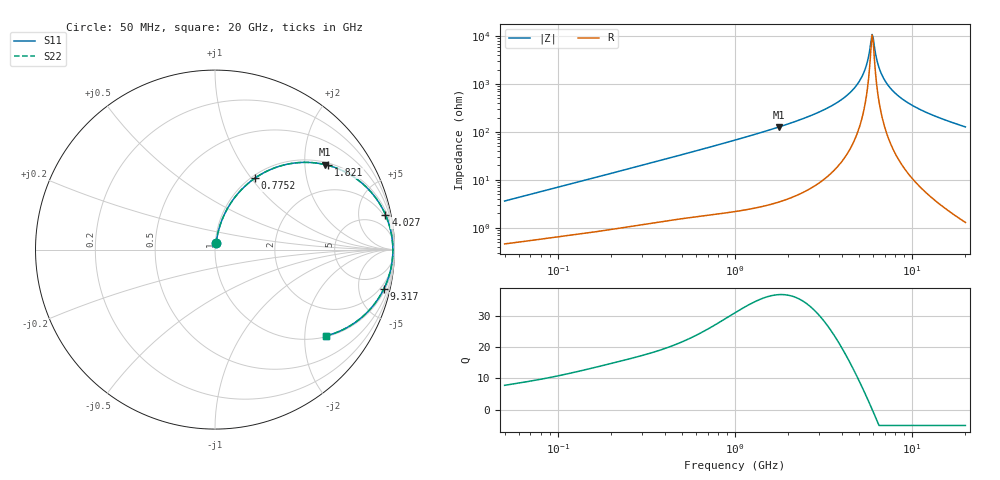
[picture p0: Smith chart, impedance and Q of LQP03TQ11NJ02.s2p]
!Murata Part Number: LQP03TQ11NJ02
!These Parameters are Measured in Series Mode Connection
!  o--[Z]--o
!Port1  Port2
!  o-------o
!Freq. Start=50[MHz] Stop=20[GHz], 401[Steps]
# Hz S RI R 50
!Freq.(Hz) S11(Real) S11(Imag) S21(Real) S21(Imag) S12(Real) S12(Imag) S22(Real) S22(Imag)
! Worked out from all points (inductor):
!   401 points, 50 MHz to 20 GHz, reference 50 ohm
!   read as one part in series: L = 11.4 nH near 51.52 MHz
!   highest Q = 36.7 at 1.767 GHz (marker M1), where L = 11.4 nH
!   self-resonance near 5.944 GHz
!   S11 on the Smith chart (normalised r, x): 50 MHz: 1.01, +0.07; 775.2 MHz: 1.04, +1.04; 1.821 GHz: 1.07, +2.63; 4.027 GHz: 1.49, +9.65; 9.317 GHz: 1.30, -8.44; 20 GHz: 1.03, -2.55
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5e7  0.00588 0.0356  0.9941 -0.0356  0.9941 -0.0356  0.00588 0.0356
1.364002e8  0.0162 0.0923  0.9838 -0.0923  0.9838 -0.0923  0.0162 0.0923
3.721004e8  0.07 0.23  0.93 -0.23  0.93 -0.23  0.07 0.23
7.751977e8  0.2215 0.3972  0.7785 -0.3972  0.7785 -0.3972  0.2215 0.3972
1e9  0.3194 0.4504  0.6806 -0.4504  0.6806 -0.4504  0.3194 0.4504
1.766834e9  0.6135 0.4735  0.3865 -0.4735  0.3865 -0.4735  0.6135 0.4735
1.820564e9  0.6299 0.4694  0.3701 -0.4694  0.3701 -0.4694  0.6299 0.4694
2.728004e9  0.8282 0.3621  0.1718 -0.3621  0.1718 -0.3621  0.8282 0.3621
4.026975e9  0.9498 0.1942  0.0502 -0.1942  0.0502 -0.1942  0.9498 0.1942
4.677679e9  0.9751 0.1215  0.0249 -0.1215  0.0249 -0.1215  0.9751 0.1215
5.194772e9  0.9857 0.0694  0.0143 -0.0694  0.0143 -0.0694  0.9857 0.0694
5.515528e9  0.9892 0.0393  0.0108 -0.0393  0.0108 -0.0393  0.9892 0.0393
5.856089e9  0.9909 0.00915  0.00915 -0.00915  0.00915 -0.00915  0.9909 0.00915
5.944466e9  0.991 0.0016  0.00903 -0.0016  0.00903 -0.0016  0.991 0.0016
6.125241e9  0.9909 -0.0135  0.00914 0.0135  0.00914 0.0135  0.9909 -0.0135
6.406762e9  0.9898 -0.0361  0.0102 0.0361  0.0102 0.0361  0.9898 -0.0361
6.601595e9  0.9885 -0.0512  0.0115 0.0512  0.0115 0.0512  0.9885 -0.0512
6.905011e9  0.9858 -0.0738  0.0142 0.0738  0.0142 0.0738  0.9858 -0.0738
7.442007e9  0.9788 -0.1112  0.0212 0.1112  0.0212 0.1112  0.9788 -0.1112
9.316812e9  0.9399 -0.2206  0.0601 0.2206  0.0601 0.2206  0.9399 -0.2206
1.295331e10  0.8336 -0.3633  0.1664 0.3633  0.1664 0.3633  0.8336 -0.3633
2e10  0.618 -0.4808  0.382 0.4808  0.382 0.4808  0.618 -0.4808
